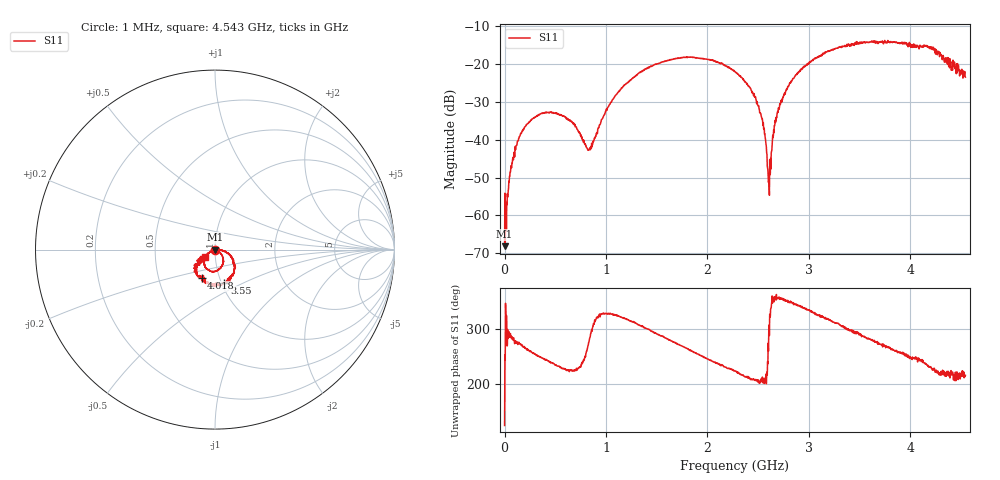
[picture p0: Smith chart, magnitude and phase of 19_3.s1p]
# HZ S RI R 50
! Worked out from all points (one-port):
!   1515 points, 1 MHz to 4.543 GHz, reference 50 ohm
!   lowest |S11| = -68.1 dB at 1 MHz (marker M1), VSWR 1.00, Z = 50 + j0.0324 ohm
!   |S11| at or under -10 dB: start of sweep to end of sweep
!   S11 on the Smith chart (normalised r, x): 1 MHz: 1.00, +0.00; 3.55 GHz: 1.03, -0.40; 4.018 GHz: 0.82, -0.27; 4.543 GHz: 0.89, -0.07
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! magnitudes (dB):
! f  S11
! 1 MHz  -68.1
! 43 MHz  -51.0
! 64 MHz  -46.8
! 160 MHz  -38.3
! 355 MHz  -33.2
! 571 MHz  -33.6
! 685 MHz  -36.0
! 835 MHz  -42.5
! 1.015 GHz  -31.6
! 1.138 GHz  -27.0
! 1.396 GHz  -21.2
! 1.705 GHz  -18.5
! 2.038 GHz  -18.9
! 2.272 GHz  -22.0
! 2.491 GHz  -30.2
! 2.554 GHz  -37.1
! 2.605 GHz  -50.6
! 2.62 GHz  -49.1
! 2.65 GHz  -38.8
! 2.68 GHz  -34.0
! 2.842 GHz  -23.8
! 3.064 GHz  -18.6
! 3.409 GHz  -15.2
! 3.55 GHz  -14.3
! 3.976 GHz  -14.7
! 4.018 GHz  -15.2
! 4.219 GHz  -16.1
! 4.543 GHz  -23.4
